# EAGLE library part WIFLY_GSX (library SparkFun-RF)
Roving Networks WiFly GSX (RN-131C) Wi-Fi Module The WiFly GSX (RN-131C) module is a complete ultra low power embedded TCP/IP solution. The WiFly GSX module is a stand alone, embedded wireless 802.11b/g networking module. SparkFun Products WiFly GSX 802.11b/g Serial Module - Roving Networks (WRL-10004)
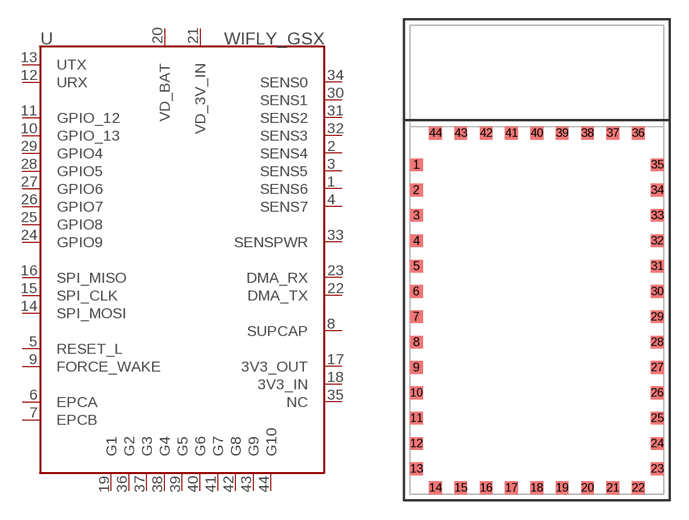
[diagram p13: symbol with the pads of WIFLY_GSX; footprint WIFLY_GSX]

Designator prefix -

## WIFLY_GSX (PROD_ID: IC-12671; SF_ID: WRL-13525)  [WIFLY_GSX]
1  SENS6
2  SENS4
3  SENS5
4  SENS7
5  RESET_L
6  EPCA
7  EPCB
8  SUPCAP
9  FORCE_WAKE
10  GPIO_13
11  GPIO_12
12  URX
13  UTX
14  SPI_MOSI
15  SPI_CLK
16  SPI_MISO
17  3V3_OUT
18  3V3_IN
19  G1
20  VD_BAT
21  VD_3V_IN
22  DMA_TX
23  DMA_RX
24  GPIO9
25  GPIO8
26  GPIO7
27  GPIO6
28  GPIO5
29  GPIO4
30  SENS1
31  SENS2
32  SENS3
33  SENSPWR
34  SENS0
35  NC
36  G2
37  G3
38  G4
39  G5
40  G6
41  G7
42  G8
43  G9
44  G10

## Footprint WIFLY_GSX (pad centres in mm)
Roving Networks RN-131C (WiFly GSX) 802.11b/g Module Wi-Fi module with a 37 x 28.5 x 3.5 mm footprint. Datasheet SparkFun Product Link
smd 1 x 1: 1 0.5,26; 2 0.5,24; 3 0.5,22; 4 0.5,20; 5 0.5,18; 6 0.5,16; 7 0.5,14; 8 0.5,12; 9 0.5,10; 10 0.5,8; 11 0.5,6; 12 0.5,4; 13 0.5,2; 14 2,0.5; 15 4,0.5; 16 6,0.5; 17 8,0.5; 18 10,0.5; 19 12,0.5; 20 14,0.5; 21 16,0.5; 22 18,0.5; 23 19.5,2; 24 19.5,4; 25 19.5,6; 26 19.5,8; 27 19.5,10; 28 19.5,12; 29 19.5,14; 30 19.5,16; 31 19.5,18; 32 19.5,20; 33 19.5,22; 34 19.5,24; 35 19.5,26; 36 18,28.5; 37 16,28.5; 38 14,28.5; 39 12,28.5; 40 10,28.5; 41 8,28.5; 42 6,28.5; 43 4,28.5; 44 2,28.5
